PROGRAM MAIN
VAR
	axis1,axis2,axis3:axis_ref;

	t:INT;
	Pos_arr1,Pos_arr2: ARRAY [0..999,1..3] OF LREAL;

	XmlSrvWrite: FB_XmlSrvWrite;
	sfilepath: T_MaxString:='E:\Test3.xml';
	sXPath: T_MaxString:='/dataentry/MAIN.Pos_arr1';
	writh_do: BOOL;
	XmlSrvRead: FB_XmlSrvRead;
	read_do: BOOL;	
		
	FiFo_GetDimension: FiFoGetDimension;
	fifo_display: STRING(255);

	FiFo_GroupIntegrate1,FiFo_GroupIntegrate2,FiFo_GroupIntegrate3: FiFoGroupIntegrate;
	FiFo_SetChannelOverride: FiFoSetChannelOverride;
	FiFo_Groupout1,FiFo_Groupout2,FiFo_Groupout3,FiFo_Disintegrate,FiFo_Override_output:st_mcoutputs;
	integrate_do: BOOL;	
	FiFo_GroupDisintegrate: FiFoGroupDisintegrate;	
	
	FiFo_Start: FiFoStart;
	start_do: BOOL;
	FiFo_Stop: FiFoStop;
	stop_do: BOOL;
	fifo_startoutput,fifo_stopoutput:st_mcoutputs;	

	FiFo_Write:FiFoWrite;
	FIFO_write_do: BOOL;
	FiFo_overWrite: FiFoOverwrite;
	FIFO_overwrite_do: BOOL;
	FIFO_write_output:st_mcoutputs;
END_VAR

IF FiFo_GetDimension.iNoOfAxes=3 AND FiFo_GetDimension.iNoOfFifoEntries=1000 THEN
	fifo_display:='Set Parameters Successfully,Please Continue';
ELSE
	fifo_display:='Please,Check Parameters';
END_IF

fifo();
fifo_pos();
power();
XML_write_read();

ACTION fifo:
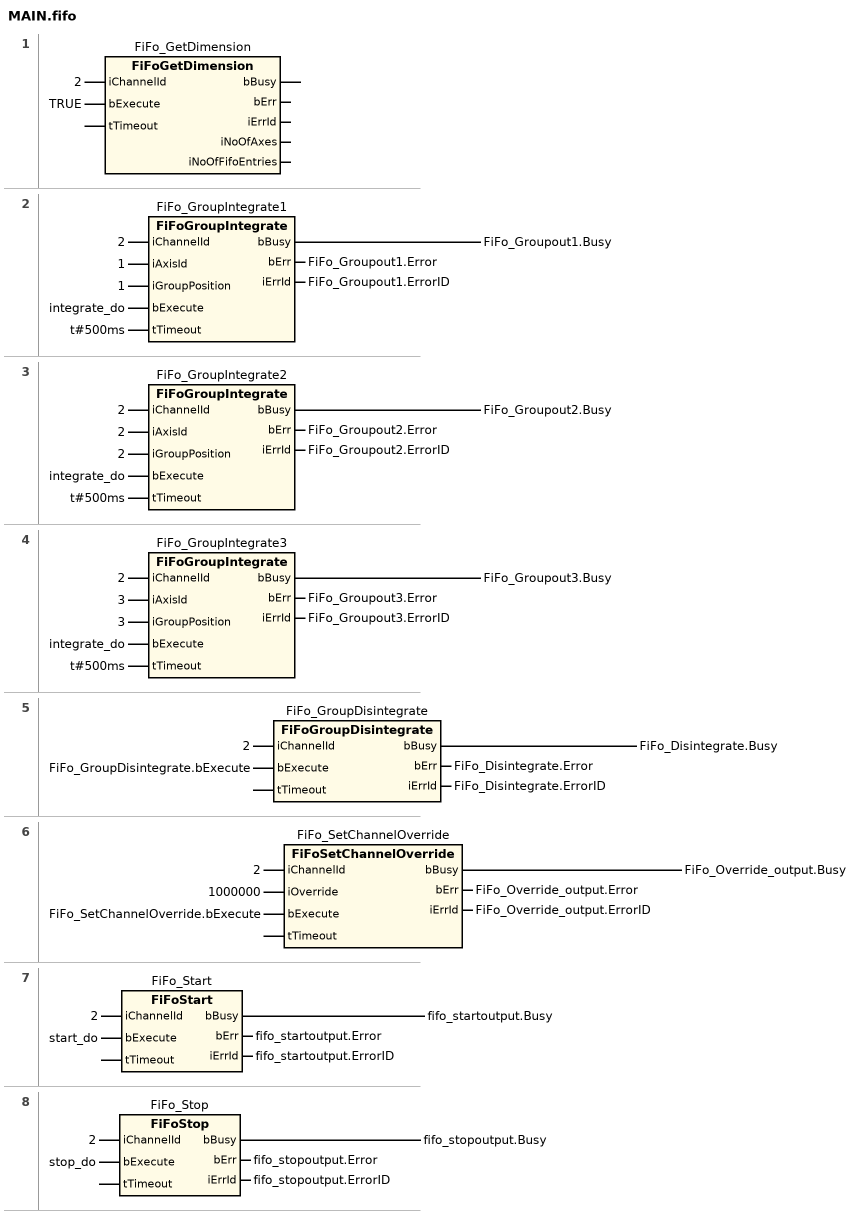
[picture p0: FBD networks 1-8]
// NETWORK 1
FiFo_GetDimension(iChannelId := 2, bExecute := TRUE); // FiFoGetDimension

// NETWORK 2
FiFo_GroupIntegrate1(
    iChannelId := 2,
    iAxisId := 1,
    iGroupPosition := 1,
    bExecute := integrate_do,
    tTimeout := t#500ms,
    bErr => FiFo_Groupout1.Error,
    iErrId => FiFo_Groupout1.ErrorID); // FiFoGroupIntegrate
FiFo_Groupout1.Busy := FiFo_GroupIntegrate1.bBusy;

// NETWORK 3
FiFo_GroupIntegrate2(
    iChannelId := 2,
    iAxisId := 2,
    iGroupPosition := 2,
    bExecute := integrate_do,
    tTimeout := t#500ms,
    bErr => FiFo_Groupout2.Error,
    iErrId => FiFo_Groupout2.ErrorID); // FiFoGroupIntegrate
FiFo_Groupout2.Busy := FiFo_GroupIntegrate2.bBusy;

// NETWORK 4
FiFo_GroupIntegrate3(
    iChannelId := 2,
    iAxisId := 3,
    iGroupPosition := 3,
    bExecute := integrate_do,
    tTimeout := t#500ms,
    bErr => FiFo_Groupout3.Error,
    iErrId => FiFo_Groupout3.ErrorID); // FiFoGroupIntegrate
FiFo_Groupout3.Busy := FiFo_GroupIntegrate3.bBusy;

// NETWORK 5
FiFo_GroupDisintegrate(
    iChannelId := 2,
    bExecute := FiFo_GroupDisintegrate.bExecute,
    bErr => FiFo_Disintegrate.Error,
    iErrId => FiFo_Disintegrate.ErrorID); // FiFoGroupDisintegrate
FiFo_Disintegrate.Busy := FiFo_GroupDisintegrate.bBusy;

// NETWORK 6
FiFo_SetChannelOverride(
    iChannelId := 2,
    iOverride := 1000000,
    bExecute := FiFo_SetChannelOverride.bExecute,
    bErr => FiFo_Override_output.Error,
    iErrId => FiFo_Override_output.ErrorID); // FiFoSetChannelOverride
FiFo_Override_output.Busy := FiFo_SetChannelOverride.bBusy;

// NETWORK 7
FiFo_Start(
    iChannelId := 2,
    bExecute := start_do,
    bErr => fifo_startoutput.Error,
    iErrId => fifo_startoutput.ErrorID); // FiFoStart
fifo_startoutput.Busy := FiFo_Start.bBusy;

// NETWORK 8
FiFo_Stop(
    iChannelId := 2,
    bExecute := stop_do,
    bErr => fifo_stopoutput.Error,
    iErrId => fifo_stopoutput.ErrorID); // FiFoStop
fifo_stopoutput.Busy := FiFo_Stop.bBusy;

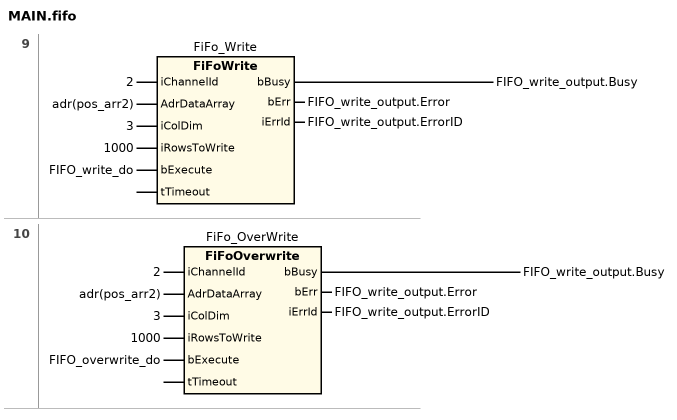
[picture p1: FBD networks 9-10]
// NETWORK 9
FiFo_Write(
    iChannelId := 2,
    AdrDataArray := adr(pos_arr2),
    iColDim := 3,
    iRowsToWrite := 1000,
    bExecute := FIFO_write_do,
    bErr => FIFO_write_output.Error,
    iErrId => FIFO_write_output.ErrorID); // FiFoWrite
FIFO_write_output.Busy := FiFo_Write.bBusy;

// NETWORK 10
FiFo_OverWrite(
    iChannelId := 2,
    AdrDataArray := adr(pos_arr2),
    iColDim := 3,
    iRowsToWrite := 1000,
    bExecute := FIFO_overwrite_do,
    bErr => FIFO_write_output.Error,
    iErrId => FIFO_write_output.ErrorID); // FiFoOverwrite
FIFO_write_output.Busy := FiFo_OverWrite.bBusy;
END_ACTION

ACTION fifo_pos:
FOR t:=0 TO 999 BY 1 DO
	Pos_arr1[t,1]:=10*SIN(0.02*t) + 2*COS(0.04*t) + 3*COS(0.02*t) - 5*COS(0.04*t);
	Pos_arr1[t,2]:=10*SIN(0.01*t) + 2*COS(0.002*t) + 3*COS(0.001*t) - 5*COS(0.02*t);
	Pos_arr1[t,3]:=10*SIN(0.03*t) + 2*COS(0.06*t) + 3*COS(0.03*t) - 5*COS(0.06*t);
END_FOR
END_ACTION

ACTION power:
axis1.PlcToNc.ControlDWord:=7;
axis2.PlcToNc.ControlDWord:=7;
axis3.PlcToNc.ControlDWord:=7;
axis1.PlcToNc.Override:=1000000;
axis2.PlcToNc.Override:=1000000;
axis3.PlcToNc.Override:=1000000;
END_ACTION

ACTION XML_write_read:
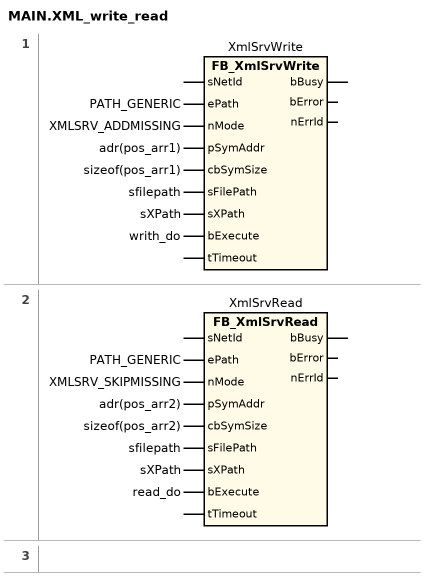
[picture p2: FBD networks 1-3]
// NETWORK 1
XmlSrvWrite(
    ePath := PATH_GENERIC,
    nMode := XMLSRV_ADDMISSING,
    pSymAddr := adr(pos_arr1),
    cbSymSize := sizeof(pos_arr1),
    sFilePath := sfilepath,
    sXPath := sXPath,
    bExecute := writh_do); // FB_XmlSrvWrite

// NETWORK 2
XmlSrvRead(
    ePath := PATH_GENERIC,
    nMode := XMLSRV_SKIPMISSING,
    pSymAddr := adr(pos_arr2),
    cbSymSize := sizeof(pos_arr2),
    sFilePath := sfilepath,
    sXPath := sXPath,
    bExecute := read_do); // FB_XmlSrvRead

// NETWORK 3
END_ACTION

END_PROGRAM
